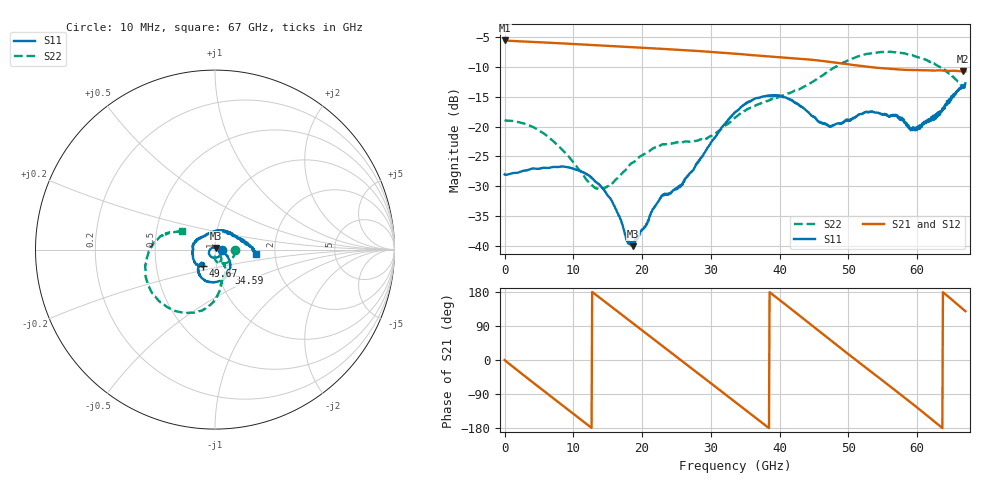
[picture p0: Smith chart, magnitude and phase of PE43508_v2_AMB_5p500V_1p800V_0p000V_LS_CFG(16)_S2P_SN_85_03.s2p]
!Keysight Technologies,N5227A,US51270237,A.10.43.00
!Date: Wednesday, August 22, 2018 17:08:12
!Correction: S11(Full 2 Port(1,3))
!S31(Full 2 Port(1,3))
!S13(Full 2 Port(1,3))
!S33(Full 2 Port(1,3))
!S2P File: Measurements: S11, S31, S13, S33:
# Hz S  dB  R 50
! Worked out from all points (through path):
!   801 points, 10 MHz to 67 GHz, reference 50 ohm
!   highest |S21| = -5.52 dB at 10 MHz (marker M1); lowest = -10.7 dB at 66.67 GHz (marker M2)
!   group delay of S21, straight-line fit = 39.2 ps
!   lowest |S11| = -40.1 dB at 18.68 GHz (marker M3), VSWR 1.02, Z = 50.3 + j0.957 ohm
!   |S11| at or under -10 dB: start of sweep to end of sweep
!   |S22| runs from -30.5 to -7.4 dB; largest |S21 - S12| = 0.0032
!   S11 on the Smith chart (normalised r, x): 10 MHz: 1.08, -0.00; 34.59 GHz: 1.12, -0.30; 49.67 GHz: 0.86, -0.16; 67 GHz: 1.60, -0.08
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1e7  -28.01 -0.8  -5.52 -0.2  -5.52 -0.2  -18.89 -0.6
2.522125e9  -27.49 -39.0  -5.68 -36.6  -5.67 -36.6  -19.37 -29.8
5.70415e9  -26.90 -80.6  -5.86 -81.7  -5.85 -81.6  -21.14 -62.9
8.300012e9  -26.70 -110.7  -6.01 -118.2  -6.00 -118.2  -23.79 -84.0
1.123082e10  -27.55 -140.1  -6.19 -159.2  -6.18 -159.2  -27.74 -92.1
1.424538e10  -30.26 -173.7  -6.37 158.7  -6.36 158.7  -30.43 -69.1
1.868346e10  -40.06 73.5  -6.66 96.8  -6.65 96.9  -25.99 -49.6
2.236791e10  -32.50 -18.4  -6.90 45.5  -6.89 45.5  -23.33 -60.2
2.47963e10  -30.51 -28.1  -7.06 11.6  -7.05 11.6  -22.73 -66.5
2.714095e10  -27.57 -25.2  -7.23 -21.2  -7.22 -21.1  -22.47 -66.8
3.040671e10  -22.09 -28.0  -7.49 -67.0  -7.48 -66.9  -21.33 -59.7
3.3505e10  -17.62 -50.4  -7.75 -110.5  -7.74 -110.4  -18.49 -61.0
3.459359e10  -16.51 -59.7  -7.84 -125.8  -7.84 -125.7  -17.55 -63.0
3.928289e10  -14.75 -101.9  -8.27 168.3  -8.26 168.4  -15.24 -75.8
4.472582e10  -18.18 -136.0  -8.77 90.8  -8.75 90.8  -12.52 -84.3
4.966634e10  -18.82 -125.9  -9.47 19.9  -9.46 19.8  -9.01 -104.3
5.251341e10  -17.58 -141.3  -9.91 -20.2  -9.90 -20.3  -7.82 -122.2
5.586291e10  -18.35 180.0  -10.25 -67.0  -10.27 -67.3  -7.42 -145.0
5.937989e10  -20.10 118.0  -10.49 -116.7  -10.51 -116.9  -8.06 -167.8
6.205949e10  -18.35 61.9  -10.57 -155.8  -10.60 -155.9  -9.21 174.5
6.666505e10  -13.47 -2.3  -10.73 133.9  -10.78 134.3  -13.23 152.4
6.7e10  -12.72 -5.6  -10.72 128.7  -10.77 128.9  -13.54 150.3
